|Texas Instruments Incorporated
|XWR6243
[IBIS Ver]   4.1
[File name]   xwr6243_v1.ibs
[Date]   06/24/2022
[File Rev]   1.0
[Source]
| Texas Instruments Incorporated.
| Analog-eLab Design Center, HPA
| 12500 TI Blvd
| Dallas, TX -75243
[Notes]   Revision History:
| Rev 1.0: 06/24/2022
| - Initial version of the model
|   Model names with a trailing _1p8 contain the model for 1.8V operation.
|   Model names with a trailing _3p3 contain the model for 3.3V operation.
| - C_comp although listed in numerical order of value are
|   obtained from varying PVT conditions. For PVT conditions for
|   each specific value refer the buffer description under
|   respective [Model]. IBIS model user is responsible for using
|   appropriate C_comp to simulate for Signal Integrity.
[Disclaimer]
| This model is designed as an aid for customers of Texas Instruments.
| TI and its licensors and suppliers make no warranties, either expressed
| or implied, with respect to this  model, including the warranties of
| merchantability or fitness for a particular purpose. The model is
| provided solely on an "as is" basis. The entire risk as to its quality
| and performance is with the customer.
| This model is subject to change without notice. Texas Instruments
| Incorporated is not responsible for updating this model.
[Copyright]
(C) Copyright 2022 Texas Instruments Incorporated.All rights reserved.
|  Component XWR6243ABGABL 161-pin FCBGA -ABL0161 package
|  Part # AWR6243ABGABLQ1/IWR6243ABGABL
[Component]   XWR6243ABGABL
[Manufacturer]   Texas Instruments
[Package]   |161 FCBGA -ABL0161 package
|  variable   typ   min   max
R_pkg   0.05   0.04   0.06
L_pkg   1.0nH   0.8nH   1.2nH
C_pkg   0.2pF   0.16pF   0.24pF
[Pin]   signal_name   model_name   R_pin   L_pin   C_pin
A1   VSSA   GND   NA   NA   NA
A2   VOUT_PA   NC   NA   NA   NA
A3   VSSA   GND   NA   NA   NA
A5   VSSA   GND   NA   NA   NA
A7   VSSA   GND   NA   NA   NA
A9   VSSA   GND   NA   NA   NA
A10   VOUT_14APLL   NC   NA   NA   NA
A13   VOUT_14SYNTH   NC   NA   NA   NA
A14   OSC_CLKOUT   OUT   NA   NA   NA
A15   VSSA   GND   NA   NA   NA
B1   FM_CW_SYNCIN1   NC   NA   NA   NA
B2   VOUT_PA   NC   NA   NA   NA
B3   VSSA   GND   NA   NA   NA
B4   TX1   NC   NA   NA   NA
B5   VSSA   GND   NA   NA   NA
B6   TX2   NC   NA   NA   NA
B7   VSSA   GND   NA   NA   NA
B8   TX3   NC   NA   NA   NA
B9   VSSA   GND   NA   NA   NA
B10   VBGAP   NC   NA   NA   NA
B11   VIN_18CLK   POWER   NA   NA   NA
B12   VIN_18VCO   POWER   NA   NA   NA
B13   VSSA   GND   NA   NA   NA
B14   VSSA   GND   NA   NA   NA
B15   FM_CW_CLKOUT   NC   NA   NA   NA
C1   VSSA   GND   NA   NA   NA
C2   VIN_13RF2   POWER   NA   NA   NA
C3   VSSA   GND   NA   NA   NA
C4   VSSA   GND   NA   NA   NA
C5   VSSA   GND   NA   NA   NA
C6   VSSA   GND   NA   NA   NA
C7   VSSA   GND   NA   NA   NA
C8   VSSA   GND   NA   NA   NA
C9   VSSA   GND   NA   NA   NA
C13   ANAMUX/GPADC5   NC   NA   NA   NA
C14   VSENSE/GPADC6   NC   NA   NA   NA
C15   VSSA   GND   NA   NA   NA
D1   FM_CW_SYNCOUT   NC   NA   NA   NA
D2   VIN_13RF2   POWER   NA   NA   NA
D13   VIOIN_18DIFF   POWER   NA   NA   NA
D15   FM_CW_SYNCIN2   NC   NA   NA   NA
E1   VSSA   GND   NA   NA   NA
E2   VSSA   GND   NA   NA   NA
E3   VSSA   GND   NA   NA   NA
E5   VSS   GND   NA   NA   NA
E6   VSS   GND   NA   NA   NA
E8   VSS   GND   NA   NA   NA
E10   VSS   GND   NA   NA   NA
E11   VSS   GND   NA   NA   NA
E13   VSSA   GND   NA   NA   NA
E14   CLKP   NC   NA   NA   NA
E15   VSSA   GND   NA   NA   NA
F2   RX4   NC   NA   NA   NA
F3   VSSA   GND   NA   NA   NA
F5   VIN_18BB   POWER   NA   NA   NA
F9   VSS   GND   NA   NA   NA
F11   VSS   GND   NA   NA   NA
F13   VDDIN   POWER   NA   NA   NA
F14   CLKM   NC   NA   NA   NA
G1   VSSA   GND   NA   NA   NA
G2   VSSA   GND   NA   NA   NA
G3   VSSA   GND   NA   NA   NA
G5   VIN_13RF1   POWER   NA   NA   NA
G6   VSS   GND   NA   NA   NA
G7   VSS   GND   NA   NA   NA
G8   VSS   GND   NA   NA   NA
G10   VSS   GND   NA   NA   NA
G13   Reserved   POWER   NA   NA   NA
G14   CSI2_TXM[0]   ODF1   NA   NA   NA
G15   CSI2_TXP[0]   ODF1   NA   NA   NA
H2   RX3   NC   NA   NA   NA
H3   VSSA   GND   NA   NA   NA
H5   VIN_13RF1   POWER   NA   NA   NA
H7   VSS   GND   NA   NA   NA
H9   VSS   GND   NA   NA   NA
H11   VSS   GND   NA   NA   NA
H13   TDI   IO2   NA   NA   NA
H14   CSI2_TXM[1]   ODF2   NA   NA   NA
H15   CSI2_TXP[1]   ODF2   NA   NA   NA
J1   VSSA   GND   NA   NA   NA
J2   VSSA   GND   NA   NA   NA
J3   VSSA   GND   NA   NA   NA
J5   VIN_13RF1   POWER   NA   NA   NA
J6   VSS   GND   NA   NA   NA
J7   VSS   GND   NA   NA   NA
J8   VSS   GND   NA   NA   NA
J10   VSS   GND   NA   NA   NA
J13   TDO   IO2   NA   NA   NA
J14   CSI2_CLKM   ODF1   NA   NA   NA
J15   CSI2_CLKP   ODF1   NA   NA   NA
K2   RX2   NC   NA   NA   NA
K3   VSSA   GND   NA   NA   NA
K5   VIN_18BB   POWER   NA   NA   NA
K7   VSS   GND   NA   NA   NA
K8   VSS   GND   NA   NA   NA
K9   VSS   GND   NA   NA   NA
K10   VSS   GND   NA   NA   NA
K11   VSS   GND   NA   NA   NA
K13   VIOIN_18   POWER   NA   NA   NA
K14   CSI2_TXM[2]   ODF2   NA   NA   NA
K15   CSI2_TXP[2]   ODF2   NA   NA   NA
L1   VSSA   GND   NA   NA   NA
L2   VSSA   GND   NA   NA   NA
L3   VSSA   GND   NA   NA   NA
L5   VSS   GND   NA   NA   NA
L6   VSS   GND   NA   NA   NA
L8   VSS   GND   NA   NA   NA
L10   VSS   GND   NA   NA   NA
L13   TMS   IO2   NA   NA   NA
L14   CSI2_TXM[3]   ODF2   NA   NA   NA
L15   CSI2_TXP[3]   ODF2   NA   NA   NA
M2   RX1   NC   NA   NA   NA
M3   VSSA   GND   NA   NA   NA
M13   TCK   IO2   NA   NA   NA
M14   HS_M_Debug1   NC   NA   NA   NA
M15   HS_P_Debug1   NC   NA   NA   NA
N1   VSSA   GND   NA   NA   NA
N2   VSSA   GND   NA   NA   NA
N3   VSSA   GND   NA   NA   NA
N4   GPIO[0]   IO1   NA   NA   NA
N5   RS232_RX   IO1   NA   NA   NA
N6   RS232_TX   IO1   NA   NA   NA
N7   GPIO[1]   IO1   NA   NA   NA
N8   NERROR_OUT   IOOD   NA   NA   NA
N9   MCU_CLK_OUT   IO1   NA   NA   NA
N10   SYNC_IN   IO2   NA   NA   NA
N11   VDDIN   POWER   NA   NA   NA
N12   WARM_RESET   IOOD   NA   NA   NA
N13   GPIO[2]   IO2   NA   NA   NA
N14   HS_M_Debug2   NC   NA   NA   NA
N15   HS_P_Debug2   NC   NA   NA   NA
P1   AnalogTest1/GPADC1  NC   NA   NA   NA
P2   AnalogTest2/GPADC2  NC   NA   NA   NA
P3   AnalogTest3/GPADC3  NC   NA   NA   NA
P4   Reserved   NC   NA   NA   NA
P5   MISO_1   IO1   NA   NA   NA
P6   SPI_HOST_INTR   NC   NA   NA   NA
P7   NERROR_IN   IOOD   NA   NA   NA
P8   QSPI_CS   IO1   NA   NA   NA
P9   QSPI[1]   IO1   NA   NA   NA
P10   QSPI[3]   IO1   NA   NA   NA
P11   SYNC_OUT   IO2   NA   NA   NA
P12   NRESET   NC   NA   NA   NA
P13   PMIC_CLK_OUT   IO2   NA   NA   NA
P14   VNWA   POWER   NA   NA   NA
P15   VDDIN   POWER   NA   NA   NA
R1   VSSA   GND   NA   NA   NA
R2   AnalogTest4/GPADC4  NC   NA   NA   NA
R3   Reserved   NC   NA   NA   NA
R4   Reserved   NC   NA   NA   NA
R5   Reserved   NC   NA   NA   NA
R6   VDDIN   POWER   NA   NA   NA
R7   SPI_CS_1   IO1   NA   NA   NA
R8   MOSI_1   IO1   NA   NA   NA
R9   SPI_CLK_1   IO1   NA   NA   NA
R10   QSPI_CLK   IO1   NA   NA   NA
R11   QSPI[0]   IO2   NA   NA   NA
R12   QSPI[2]   IO2   NA   NA   NA
R13   VIOIN   POWER   NA   NA   NA
R14   VIN_SRAM   POWER   NA   NA   NA
R15   VSS   GND   NA   NA   NA
[Diff Pin]   inv_pin   vdiff   tdelay_typ   tdelay_min   tdelay_max
G15   G14   0.2   NA   NA   NA
H15   H14   0.2   NA   NA   NA
J15   J14   0.2   NA   NA   NA
K15   K14   0.2   NA   NA   NA
L15   L14   0.2   NA   NA   NA
|  Component XWR6243ABGABLR 161-pin FCBGA -ABL0161 package
|  Part # AWR6243ABGABLRQ1/IWR6243ABGABLR
[Component]   XWR6243ABGABLR
[Manufacturer]   Texas Instruments
[Package]   |161 FCBGA -ABL0161 package
|  variable   typ   min   max
R_pkg   0.05   0.04   0.06
L_pkg   1.0nH   0.8nH   1.2nH
C_pkg   0.2pF   0.16pF   0.24pF
[Pin]   signal_name   model_name   R_pin   L_pin   C_pin
A1   VSSA   GND   NA   NA   NA
A2   VOUT_PA   NC   NA   NA   NA
A3   VSSA   GND   NA   NA   NA
A5   VSSA   GND   NA   NA   NA
A7   VSSA   GND   NA   NA   NA
A9   VSSA   GND   NA   NA   NA
A10   VOUT_14APLL   NC   NA   NA   NA
A13   VOUT_14SYNTH   NC   NA   NA   NA
A14   OSC_CLKOUT   OUT   NA   NA   NA
A15   VSSA   GND   NA   NA   NA
B1   FM_CW_SYNCIN1   NC   NA   NA   NA
B2   VOUT_PA   NC   NA   NA   NA
B3   VSSA   GND   NA   NA   NA
B4   TX1   NC   NA   NA   NA
B5   VSSA   GND   NA   NA   NA
B6   TX2   NC   NA   NA   NA
B7   VSSA   GND   NA   NA   NA
B8   TX3   NC   NA   NA   NA
B9   VSSA   GND   NA   NA   NA
B10   VBGAP   NC   NA   NA   NA
B11   VIN_18CLK   POWER   NA   NA   NA
B12   VIN_18VCO   POWER   NA   NA   NA
B13   VSSA   GND   NA   NA   NA
B14   VSSA   GND   NA   NA   NA
B15   FM_CW_CLKOUT   NC   NA   NA   NA
C1   VSSA   GND   NA   NA   NA
C2   VIN_13RF2   POWER   NA   NA   NA
C3   VSSA   GND   NA   NA   NA
C4   VSSA   GND   NA   NA   NA
C5   VSSA   GND   NA   NA   NA
C6   VSSA   GND   NA   NA   NA
C7   VSSA   GND   NA   NA   NA
C8   VSSA   GND   NA   NA   NA
C9   VSSA   GND   NA   NA   NA
C13   ANAMUX/GPADC5   NC   NA   NA   NA
C14   VSENSE/GPADC6   NC   NA   NA   NA
C15   VSSA   GND   NA   NA   NA
D1   FM_CW_SYNCOUT   NC   NA   NA   NA
D2   VIN_13RF2   POWER   NA   NA   NA
D13   VIOIN_18DIFF   POWER   NA   NA   NA
D15   FM_CW_SYNCIN2   NC   NA   NA   NA
E1   VSSA   GND   NA   NA   NA
E2   VSSA   GND   NA   NA   NA
E3   VSSA   GND   NA   NA   NA
E5   VSS   GND   NA   NA   NA
E6   VSS   GND   NA   NA   NA
E8   VSS   GND   NA   NA   NA
E10   VSS   GND   NA   NA   NA
E11   VSS   GND   NA   NA   NA
E13   VSSA   GND   NA   NA   NA
E14   CLKP   NC   NA   NA   NA
E15   VSSA   GND   NA   NA   NA
F2   RX4   NC   NA   NA   NA
F3   VSSA   GND   NA   NA   NA
F5   VIN_18BB   POWER   NA   NA   NA
F9   VSS   GND   NA   NA   NA
F11   VSS   GND   NA   NA   NA
F13   VDDIN   POWER   NA   NA   NA
F14   CLKM   NC   NA   NA   NA
G1   VSSA   GND   NA   NA   NA
G2   VSSA   GND   NA   NA   NA
G3   VSSA   GND   NA   NA   NA
G5   VIN_13RF1   POWER   NA   NA   NA
G6   VSS   GND   NA   NA   NA
G7   VSS   GND   NA   NA   NA
G8   VSS   GND   NA   NA   NA
G10   VSS   GND   NA   NA   NA
G13   Reserved   POWER   NA   NA   NA
G14   CSI2_TXM[0]   ODF1   NA   NA   NA
G15   CSI2_TXP[0]   ODF1   NA   NA   NA
H2   RX3   NC   NA   NA   NA
H3   VSSA   GND   NA   NA   NA
H5   VIN_13RF1   POWER   NA   NA   NA
H7   VSS   GND   NA   NA   NA
H9   VSS   GND   NA   NA   NA
H11   VSS   GND   NA   NA   NA
H13   TDI   IO2   NA   NA   NA
H14   CSI2_TXM[1]   ODF2   NA   NA   NA
H15   CSI2_TXP[1]   ODF2   NA   NA   NA
J1   VSSA   GND   NA   NA   NA
J2   VSSA   GND   NA   NA   NA
J3   VSSA   GND   NA   NA   NA
J5   VIN_13RF1   POWER   NA   NA   NA
J6   VSS   GND   NA   NA   NA
J7   VSS   GND   NA   NA   NA
J8   VSS   GND   NA   NA   NA
J10   VSS   GND   NA   NA   NA
J13   TDO   IO2   NA   NA   NA
J14   CSI2_CLKM   ODF1   NA   NA   NA
J15   CSI2_CLKP   ODF1   NA   NA   NA
K2   RX2   NC   NA   NA   NA
K3   VSSA   GND   NA   NA   NA
K5   VIN_18BB   POWER   NA   NA   NA
K7   VSS   GND   NA   NA   NA
K8   VSS   GND   NA   NA   NA
K9   VSS   GND   NA   NA   NA
K10   VSS   GND   NA   NA   NA
K11   VSS   GND   NA   NA   NA
K13   VIOIN_18   POWER   NA   NA   NA
K14   CSI2_TXM[2]   ODF2   NA   NA   NA
K15   CSI2_TXP[2]   ODF2   NA   NA   NA
L1   VSSA   GND   NA   NA   NA
L2   VSSA   GND   NA   NA   NA
L3   VSSA   GND   NA   NA   NA
L5   VSS   GND   NA   NA   NA
L6   VSS   GND   NA   NA   NA
L8   VSS   GND   NA   NA   NA
L10   VSS   GND   NA   NA   NA
L13   TMS   IO2   NA   NA   NA
L14   CSI2_TXM[3]   ODF2   NA   NA   NA
L15   CSI2_TXP[3]   ODF2   NA   NA   NA
M2   RX1   NC   NA   NA   NA
M3   VSSA   GND   NA   NA   NA
M13   TCK   IO2   NA   NA   NA
M14   HS_M_Debug1   NC   NA   NA   NA
M15   HS_P_Debug1   NC   NA   NA   NA
N1   VSSA   GND   NA   NA   NA
N2   VSSA   GND   NA   NA   NA
N3   VSSA   GND   NA   NA   NA
N4   GPIO[0]   IO1   NA   NA   NA
N5   RS232_RX   IO1   NA   NA   NA
N6   RS232_TX   IO1   NA   NA   NA
N7   GPIO[1]   IO1   NA   NA   NA
N8   NERROR_OUT   IOOD   NA   NA   NA
N9   MCU_CLK_OUT   IO1   NA   NA   NA
N10   SYNC_IN   IO2   NA   NA   NA
N11   VDDIN   POWER   NA   NA   NA
N12   WARM_RESET   IOOD   NA   NA   NA
N13   GPIO[2]   IO2   NA   NA   NA
N14   HS_M_Debug2   NC   NA   NA   NA
N15   HS_P_Debug2   NC   NA   NA   NA
P1   AnalogTest1/GPADC1  NC   NA   NA   NA
P2   AnalogTest2/GPADC2  NC   NA   NA   NA
P3   AnalogTest3/GPADC3  NC   NA   NA   NA
P4   Reserved   NC   NA   NA   NA
P5   MISO_1   IO1   NA   NA   NA
P6   SPI_HOST_INTR   NC   NA   NA   NA
P7   NERROR_IN   IOOD   NA   NA   NA
P8   QSPI_CS   IO1   NA   NA   NA
P9   QSPI[1]   IO1   NA   NA   NA
P10   QSPI[3]   IO1   NA   NA   NA
P11   SYNC_OUT   IO2   NA   NA   NA
P12   NRESET   NC   NA   NA   NA
P13   PMIC_CLK_OUT   IO2   NA   NA   NA
P14   VNWA   POWER   NA   NA   NA
P15   VDDIN   POWER   NA   NA   NA
R1   VSSA   GND   NA   NA   NA
R2   AnalogTest4/GPADC4  NC   NA   NA   NA
R3   Reserved   NC   NA   NA   NA
R4   Reserved   NC   NA   NA   NA
R5   Reserved   NC   NA   NA   NA
R6   VDDIN   POWER   NA   NA   NA
R7   SPI_CS_1   IO1   NA   NA   NA
R8   MOSI_1   IO1   NA   NA   NA
R9   SPI_CLK_1   IO1   NA   NA   NA
R10   QSPI_CLK   IO1   NA   NA   NA
R11   QSPI[0]   IO2   NA   NA   NA
R12   QSPI[2]   IO2   NA   NA   NA
R13   VIOIN   POWER   NA   NA   NA
R14   VIN_SRAM   POWER   NA   NA   NA
R15   VSS   GND   NA   NA   NA
[Diff Pin]   inv_pin   vdiff   tdelay_typ   tdelay_min   tdelay_max
G15   G14   0.2   NA   NA   NA
H15   H14   0.2   NA   NA   NA
J15   J14   0.2   NA   NA   NA
K15   K14   0.2   NA   NA   NA
L15   L14   0.2   NA   NA   NA
| Model IOOD
[Model Selector] IOOD
|SC1 IS A SLEW RATE CONTROL PIN
|5% SUPPLY VARIATION MODES WITH 1.8V NOM SUPPLY
IOOD_V_PUPDOFF_5P_SC1_1P8  Cell operated at 1.8(nom)
|IOOD_V_PUPDOFF_5P_SC1_1P8; BUFFER WITH WEAK PULUP/PULLDOWN OFF AT 5% SUPPLY
|VARIATION WITH SC1=1 MEANING SLOW MODE OF OPERATION
IOOD_V_PD_ON_5P_!SC1_1P8  Cell operated at 1.8(nom)
|IOOD_V_PD_ON_5P_!SC1_1P8; BUFFER WITH WEAK_PULLDOWN_ON AT 5% SUPPLY
|VARIATION WITH SC1=0 MEANING FAST MODE OF OPERATION
IOOD_V_PD_ON_5P_SC1_1P8  Cell operated at 1.8(nom)
|IOOD_V_PD_ON_5P_SC1_1P8; BUFFER WITH WEAK_PULLDOWN_ON AT 5% SUPPLY
|VARIATION WITH SC1=1 MEANING SLOW MODE OF OPERATION
IOOD_V_PU_ON_5P_!SC1_1P8  Cell operated at 1.8(nom)
|IOOD_V_PU_ON_5P_!SC1_1P8; BUFFER WITH WEAK_PULLUP_ON AT 5% SUPPLY
|VARIATION WITH SC1=0 MEANING FAST MODE OF OPERATION
IOOD_V_PUPDOFF_5P_!SC1_1P8  Cell operated at 1.8(nom)
|IOOD_V_PUPDOFF_5P_!SC1_1P8; BUFFER WITH WEAK PULUP/PULLDOWN OFF AT 5% SUPPLY
|VARIATION WITH SC1=0 MEANING FAST MODE OF OPERATION
IOOD_V_PU_ON_5P_SC1_1P8  Cell operated at 1.8(nom)
|IOOD_V_PU_ON_5P_SC1_1P8; BUFFER WITH WEAK_PULLUP_ON AT 5% SUPPLY
|VARIATION WITH SC1=1 MEANING SLOW MODE OF OPERATION
|5% SUPPLY VARIATION MODES WITH 3.3V NOM SUPPLY
IOOD_V_PUPDOFF_5P_SC1_3P3  Cell operated at 3.3(nom)
|IOOD_V_PUPDOFF_5P_SC1_3P3; BUFFER WITH WEAK PULUP/PULLDOWN OFF AT 5% SUPPLY
|VARIATION WITH SC1=1 MEANING SLOW MODE OF OPERATION
IOOD_V_PD_ON_5P_!SC1_3P3  Cell operated at 3.3(nom)
|IOOD_V_PD_ON_5P_!SC1_3P3; BUFFER WITH WEAK_PULLDOWN_ON AT 5% SUPPLY
|VARIATION WITH SC1=0 MEANING FAST MODE OF OPERATION
IOOD_V_PD_ON_5P_SC1_3P3  Cell operated at 3.3(nom)
|IOOD_V_PD_ON_5P_SC1_3P3; BUFFER WITH WEAK_PULLDOWN_ON AT 5% SUPPLY
|VARIATION WITH SC1=1 MEANING SLOW MODE OF OPERATION
IOOD_V_PU_ON_5P_!SC1_3P3  Cell operated at 3.3(nom)
|IOOD_V_PU_ON_5P_!SC1_3P3; BUFFER WITH WEAK_PULLUP_ON AT 5% SUPPLY
|VARIATION WITH SC1=0 MEANING FAST MODE OF OPERATION
IOOD_V_PUPDOFF_5P_!SC1_3P3  Cell operated at 3.3(nom)
|IOOD_V_PUPDOFF_5P_!SC1_3P3; BUFFER WITH WEAK PULUP/PULLDOWN OFF AT 5% SUPPLY
|VARIATION WITH SC1=0 MEANING FAST MODE OF OPERATION
IOOD_V_PU_ON_5P_SC1_3P3  Cell operated at 3.3(nom)
|IOOD_V_PU_ON_5P_SC1_3P3; BUFFER WITH WEAK_PULLUP_ON AT 5% SUPPLY
|VARIATION WITH SC1=1 MEANING SLOW MODE OF OPERATION
| 10% SUPPLY VARIATION MODES WITH 1.8V NOM SUPPLY
IOOD_V_PUPDOFF_10P_SC1_1P8  Cell operated at 1.8(nom)
|IOOD_V_PUPDOFF_10P_SC1_1P8; BUFFER WITH WEAK PULUP/PULLDOWN OFF AT 10% SUPPLY
|VARIATION WITH SC1=1 MEANING SLOW MODE OF OPERATION
IOOD_V_PD_ON_10P_!SC1_1P8  Cell operated at 1.8(nom)
|IOOD_V_PD_ON_10P_!SC1_1P8; BUFFER WITH WEAK_PULLDOWN_ON AT 10% SUPPLY
|VARIATION WITH SC1=0 MEANING FAST MODE OF OPERATION
IOOD_V_PD_ON_10P_SC1_1P8  Cell operated at 1.8(nom)
|IOOD_V_PD_ON_10P_SC1_1P8; BUFFER WITH WEAK_PULLDOWN_ON AT 10% SUPPLY
|VARIATION WITH SC1=1 MEANING SLOW MODE OF OPERATION
IOOD_V_PU_ON_10P_!SC1_1P8  Cell operated at 1.8(nom)
|IOOD_V_PU_ON_10P_!SC1_1P8; BUFFER WITH WEAK_PULLUP_ON AT 10% SUPPLY
|VARIATION WITH SC1=0 MEANING FAST MODE OF OPERATION
IOOD_V_PUPDOFF_10P_!SC1_1P8  Cell operated at 1.8(nom)
|IOOD_V_PUPDOFF_10P_!SC1_1P8; BUFFER WITH WEAK PULUP/PULLDOWN OFF AT 10% SUPPLY
|VARIATION WITH SC1=0 MEANING FAST MODE OF OPERATION
IOOD_V_PU_ON_10P_SC1_1P8  Cell operated at 1.8(nom)
|IOOD_V_PU_ON_10P_SC1_1P8; BUFFER WITH WEAK_PULLUP_ON AT 10% SUPPLY
|VARIATION WITH SC1=1 MEANING SLOW MODE OF OPERATION
| 10% SUPPLY VARIATION MODES WITH 3.3V NOM SUPPLY
IOOD_V_PUPDOFF_10P_SC1_3P3  Cell operated at 3.3(nom)
|IOOD_V_PUPDOFF_10P_SC1_3P3; BUFFER WITH WEAK PULUP/PULLDOWN OFF AT 10% SUPPLY
|VARIATION WITH SC1=1 MEANING SLOW MODE OF OPERATION
IOOD_V_PD_ON_10P_!SC1_3P3  Cell operated at 3.3(nom)
|IOOD_V_PD_ON_10P_!SC1_3P3; BUFFER WITH WEAK_PULLDOWN_ON 10% SUPPLY
|VARIATION WITH SC1=0 MEANING FAST MODE OF OPERATION
IOOD_V_PD_ON_10P_SC1_3P3  Cell operated at 3.3(nom)
|IOOD_V_PD_ON_10P_SC1_3P3; BUFFER WITH WEAK_PULLDOWN_ON AT 10% SUPPLY
|VARIATION WITH SC1=1 MEANING SLOW MODE OF OPERATION
IOOD_V_PU_ON_10P_!SC1_3P3  Cell operated at 3.3(nom)
|IOOD_V_PU_ON_10P_!SC1_3P3; BUFFER WITH WEAK_PULLUP_ON AT 10% SUPPLY
|VARIATION WITH SC1=0 MEANING FAST MODE OF OPERATION
IOOD_V_PUPDOFF_10P_!SC1_3P3  Cell operated at 3.3(nom)
|IOOD_V_PUPDOFF_10P_!SC1_3P3; BUFFER WITH WEAK PULUP/PULLDOWN OFF AT 10% SUPPLY
|VARIATION WITH SC1=0 MEANING FAST MODE OF OPERATION
IOOD_V_PU_ON_10P_SC1_3P3  Cell operated at 3.3(nom)
|IOOD_V_PU_ON_10P_SC1_3P3; BUFFER WITH WEAK_PULLUP_ON AT 10% SUPPLY
|VARIATION WITH SC1=1 MEANING SLOW MODE OF OPERATION
| Model IO1
[Model Selector] IO1
|SC1 IS A SLEW RATE CONTROL PIN
|5% SUPPLY VARIATION MODES WITH 1.8V NOM SUPPLY
IO1_V_PUPDOFF_5P_SC1_1P8  Cell operated at 1.8(nom)
|IO1_V_PUPDOFF_5P_SC1_1P8; BUFFER WITH WEAK PULUP/PULLDOWN OFF AT 5% SUPPLY
|VARIATION WITH SC1=1 MEANING SLOW MODE OF OPERATION
IO1_V_PD_ON_5P_!SC1_1P8  Cell operated at 1.8(nom)
|IO1_V_PD_ON_5P_!SC1_1P8; BUFFER WITH WEAK_PULLDOWN_ON AT 5% SUPPLY
|VARIATION WITH SC1=0 MEANING FAST MODE OF OPERATION
IO1_V_PD_ON_5P_SC1_1P8  Cell operated at 1.8(nom)
|IO1_V_PD_ON_5P_SC1_1P8; BUFFER WITH WEAK_PULLDOWN_ON AT 5% SUPPLY
|VARIATION WITH SC1=1 MEANING SLOW MODE OF OPERATION
IO1_V_PU_ON_5P_!SC1_1P8  Cell operated at 1.8(nom)
|IO1_V_PU_ON_5P_!SC1_1P8; BUFFER WITH WEAK_PULLUP_ON AT 5% SUPPLY
|VARIATION WITH SC1=0 MEANING FAST MODE OF OPERATION
IO1_V_PUPDOFF_5P_!SC1_1P8  Cell operated at 1.8(nom)
|IO1_V_PUPDOFF_5P_!SC1_1P8; BUFFER WITH WEAK PULUP/PULLDOWN OFF AT 5% SUPPLY
|VARIATION WITH SC1=0 MEANING FAST MODE OF OPERATION
IO1_V_PU_ON_5P_SC1_1P8  Cell operated at 1.8(nom)
|IO1_V_PU_ON_5P_SC1_1P8; BUFFER WITH WEAK_PULLUP_ON AT 5% SUPPLY
|VARIATION WITH SC1=1 MEANING SLOW MODE OF OPERATION
|5% SUPPLY VARIATION MODES WITH 3.3V NOM SUPPLY
IO1_V_PUPDOFF_5P_SC1_3P3  Cell operated at 3.3(nom)
|IO1_V_PUPDOFF_5P_SC1_3P3; BUFFER WITH WEAK PULUP/PULLDOWN OFF AT 5% SUPPLY
|VARIATION WITH SC1=1 MEANING SLOW MODE OF OPERATION
IO1_V_PD_ON_5P_!SC1_3P3  Cell operated at 3.3(nom)
|IO1_V_PD_ON_5P_!SC1_3P3; BUFFER WITH WEAK_PULLDOWN_ON AT 5% SUPPLY
|VARIATION WITH SC1=0 MEANING FAST MODE OF OPERATION
IO1_V_PD_ON_5P_SC1_3P3  Cell operated at 3.3(nom)
|IO1_V_PD_ON_5P_SC1_3P3; BUFFER WITH WEAK_PULLDOWN_ON AT 5% SUPPLY
|VARIATION WITH SC1=1 MEANING SLOW MODE OF OPERATION
IO1_V_PU_ON_5P_!SC1_3P3  Cell operated at 3.3(nom)
|IO1_V_PU_ON_5P_!SC1_3P3; BUFFER WITH WEAK_PULLUP_ON AT 5% SUPPLY
|VARIATION WITH SC1=0 MEANING FAST MODE OF OPERATION
IO1_V_PUPDOFF_5P_!SC1_3P3  Cell operated at 3.3(nom)
|IO1_V_PUPDOFF_5P_!SC1_3P3; BUFFER WITH WEAK PULUP/PULLDOWN OFF AT 5% SUPPLY
|VARIATION WITH SC1=0 MEANING FAST MODE OF OPERATION
IO1_V_PU_ON_5P_SC1_3P3  Cell operated at 3.3(nom)
|IO1_V_PU_ON_5P_SC1_3P3; BUFFER WITH WEAK_PULLUP_ON AT 5% SUPPLY
|VARIATION WITH SC1=1 MEANING SLOW MODE OF OPERATION
| 10% SUPPLY VARIATION MODES WITH 1.8V NOM SUPPLY
IO1_V_PUPDOFF_10P_SC1_1P8  Cell operated at 1.8(nom)
|IO1_V_PUPDOFF_10P_SC1_1P8; BUFFER WITH WEAK PULUP/PULLDOWN OFF AT 10% SUPPLY
|VARIATION WITH SC1=1 MEANING SLOW MODE OF OPERATION
IO1_V_PD_ON_10P_!SC1_1P8  Cell operated at 1.8(nom)
|IO1_V_PD_ON_10P_!SC1_1P8; BUFFER WITH WEAK_PULLDOWN_ON AT 10% SUPPLY
|VARIATION WITH SC1=0 MEANING FAST MODE OF OPERATION
IO1_V_PD_ON_10P_SC1_1P8  Cell operated at 1.8(nom)
|IO1_V_PD_ON_10P_SC1_1P8; BUFFER WITH WEAK_PULLDOWN_ON AT 10% SUPPLY
|VARIATION WITH SC1=1 MEANING SLOW MODE OF OPERATION
IO1_V_PU_ON_10P_!SC1_1P8  Cell operated at 1.8(nom)
|IO1_V_PU_ON_10P_!SC1_1P8; BUFFER WITH WEAK_PULLUP_ON AT 10% SUPPLY
|VARIATION WITH SC1=0 MEANING FAST MODE OF OPERATION
IO1_V_PUPDOFF_10P_!SC1_1P8  Cell operated at 1.8(nom)
|IO1_V_PUPDOFF_10P_!SC1_1P8; BUFFER WITH WEAK PULUP/PULLDOWN OFF AT 10% SUPPLY
|VARIATION WITH SC1=0 MEANING FAST MODE OF OPERATION
IO1_V_PU_ON_10P_SC1_1P8  Cell operated at 1.8(nom)
|IO1_V_PU_ON_10P_SC1_1P8; BUFFER WITH WEAK_PULLUP_ON AT 10% SUPPLY
|VARIATION WITH SC1=1 MEANING SLOW MODE OF OPERATION
| 10% SUPPLY VARIATION MODES WITH 3.3V NOM SUPPLY
IO1_V_PUPDOFF_10P_SC1_3P3  Cell operated at 3.3(nom)
|IO1_V_PUPDOFF_10P_SC1_3P3; BUFFER WITH WEAK PULUP/PULLDOWN OFF AT 10% SUPPLY
|VARIATION WITH SC1=1 MEANING SLOW MODE OF OPERATION
IO1_V_PD_ON_10P_!SC1_3P3  Cell operated at 3.3(nom)
|IO1_V_PD_ON_10P_!SC1_3P3; BUFFER WITH WEAK_PULLDOWN_ON 10% SUPPLY
|VARIATION WITH SC1=0 MEANING FAST MODE OF OPERATION
IO1_V_PD_ON_10P_SC1_3P3  Cell operated at 3.3(nom)
|IO1_V_PD_ON_10P_SC1_3P3; BUFFER WITH WEAK_PULLDOWN_ON AT 10% SUPPLY
|VARIATION WITH SC1=1 MEANING SLOW MODE OF OPERATION
IO1_V_PU_ON_10P_!SC1_3P3  Cell operated at 3.3(nom)
|IO1_V_PU_ON_10P_!SC1_3P3; BUFFER WITH WEAK_PULLUP_ON AT 10% SUPPLY
|VARIATION WITH SC1=0 MEANING FAST MODE OF OPERATION
IO1_V_PUPDOFF_10P_!SC1_3P3  Cell operated at 3.3(nom)
|IO1_V_PUPDOFF_10P_!SC1_3P3; BUFFER WITH WEAK PULUP/PULLDOWN OFF AT 10% SUPPLY
|VARIATION WITH SC1=0 MEANING FAST MODE OF OPERATION
IO1_V_PU_ON_10P_SC1_3P3  Cell operated at 3.3(nom)
|IO1_V_PU_ON_10P_SC1_3P3; BUFFER WITH WEAK_PULLUP_ON AT 10% SUPPLY
|VARIATION WITH SC1=1 MEANING SLOW MODE OF OPERATION
| Model IO2
[Model Selector] IO2
|SC1 IS A SLEW RATE CONTROL PIN
|5% SUPPLY VARIATION MODES WITH 1.8V NOM SUPPLY
IO2_H_PUPDOFF_5P_SC1_1P8  Cell operated at 1.8(nom)
|IO2_H_PUPDOFF_5P_SC1_1P8; BUFFER WITH WEAK PULUP/PULLDOWN OFF AT 5% SUPPLY
|VARIATION WITH SC1=1 MEANING SLOW MODE OF OPERATION
IO2_H_PD_ON_5P_!SC1_1P8  Cell operated at 1.8(nom)
|IO2_H_PD_ON_5P_!SC1_1P8; BUFFER WITH WEAK_PULLDOWN_ON AT 5% SUPPLY
|VARIATION WITH SC1=0 MEANING FAST MODE OF OPERATION
IO2_H_PD_ON_5P_SC1_1P8  Cell operated at 1.8(nom)
|IO2_H_PD_ON_5P_SC1_1P8; BUFFER WITH WEAK_PULLDOWN_ON AT 5% SUPPLY
|VARIATION WITH SC1=1 MEANING SLOW MODE OF OPERATION
IO2_H_PU_ON_5P_!SC1_1P8  Cell operated at 1.8(nom)
|IO2_H_PU_ON_5P_!SC1_1P8; BUFFER WITH WEAK_PULLUP_ON AT 5% SUPPLY
|VARIATION WITH SC1=0 MEANING FAST MODE OF OPERATION
IO2_H_PUPDOFF_5P_!SC1_1P8  Cell operated at 1.8(nom)
|IO2_H_PUPDOFF_5P_!SC1_1P8; BUFFER WITH WEAK PULUP/PULLDOWN OFF AT 5% SUPPLY
|VARIATION WITH SC1=0 MEANING FAST MODE OF OPERATION
IO2_H_PU_ON_5P_SC1_1P8  Cell operated at 1.8(nom)
|IO2_H_PU_ON_5P_SC1_1P8; BUFFER WITH WEAK_PULLUP_ON AT 5% SUPPLY
|VARIATION WITH SC1=1 MEANING SLOW MODE OF OPERATION
|5% SUPPLY VARIATION MODES WITH 3.3V NOM SUPPLY
IO2_H_PUPDOFF_5P_SC1_3P3  Cell operated at 3.3(nom)
|IO2_H_PUPDOFF_5P_SC1_3P3; BUFFER WITH WEAK PULUP/PULLDOWN OFF AT 5% SUPPLY
|VARIATION WITH SC1=1 MEANING SLOW MODE OF OPERATION
IO2_H_PD_ON_5P_!SC1_3P3  Cell operated at 3.3(nom)
|IO2_H_PD_ON_5P_!SC1_3P3; BUFFER WITH WEAK_PULLDOWN_ON AT 5% SUPPLY
|VARIATION WITH SC1=0 MEANING FAST MODE OF OPERATION
IO2_H_PD_ON_5P_SC1_3P3  Cell operated at 3.3(nom)
|IO2_H_PD_ON_5P_SC1_3P3; BUFFER WITH WEAK_PULLDOWN_ON AT 5% SUPPLY
|VARIATION WITH SC1=1 MEANING SLOW MODE OF OPERATION
IO2_H_PU_ON_5P_!SC1_3P3  Cell operated at 3.3(nom)
|IO2_H_PU_ON_5P_!SC1_3P3; BUFFER WITH WEAK_PULLUP_ON AT 5% SUPPLY
|VARIATION WITH SC1=0 MEANING FAST MODE OF OPERATION
IO2_H_PUPDOFF_5P_!SC1_3P3  Cell operated at 3.3(nom)
|IO2_H_PUPDOFF_5P_!SC1_3P3; BUFFER WITH WEAK PULUP/PULLDOWN OFF AT 5% SUPPLY
|VARIATION WITH SC1=0 MEANING FAST MODE OF OPERATION
IO2_H_PU_ON_5P_SC1_3P3  Cell operated at 3.3(nom)
|IO2_H_PU_ON_5P_SC1_3P3; BUFFER WITH WEAK_PULLUP_ON AT 5% SUPPLY
|VARIATION WITH SC1=1 MEANING SLOW MODE OF OPERATION
| 10% SUPPLY VARIATION MODES WITH 1.8V NOM SUPPLY
IO2_H_PUPDOFF_10P_SC1_1P8  Cell operated at 1.8(nom)
|IO2_H_PUPDOFF_10P_SC1_1P8; BUFFER WITH WEAK PULUP/PULLDOWN OFF AT 10% SUPPLY
|VARIATION WITH SC1=1 MEANING SLOW MODE OF OPERATION
IO2_H_PD_ON_10P_!SC1_1P8  Cell operated at 1.8(nom)
|IO2_H_PD_ON_10P_!SC1_1P8; BUFFER WITH WEAK_PULLDOWN_ON AT 10% SUPPLY
|VARIATION WITH SC1=0 MEANING FAST MODE OF OPERATION
IO2_H_PD_ON_10P_SC1_1P8  Cell operated at 1.8(nom)
|IO2_H_PD_ON_10P_SC1_1P8; BUFFER WITH WEAK_PULLDOWN_ON AT 10% SUPPLY
|VARIATION WITH SC1=1 MEANING SLOW MODE OF OPERATION
IO2_H_PU_ON_10P_!SC1_1P8  Cell operated at 1.8(nom)
|IO2_H_PU_ON_10P_!SC1_1P8; BUFFER WITH WEAK_PULLUP_ON AT 10% SUPPLY
|VARIATION WITH SC1=0 MEANING FAST MODE OF OPERATION
IO2_H_PUPDOFF_10P_!SC1_1P8  Cell operated at 1.8(nom)
|IO2_H_PUPDOFF_10P_!SC1_1P8; BUFFER WITH WEAK PULUP/PULLDOWN OFF AT 10% SUPPLY
|VARIATION WITH SC1=0 MEANING FAST MODE OF OPERATION
IO2_H_PU_ON_10P_SC1_1P8  Cell operated at 1.8(nom)
|IO2_H_PU_ON_10P_SC1_1P8; BUFFER WITH WEAK_PULLUP_ON AT 10% SUPPLY
|VARIATION WITH SC1=1 MEANING SLOW MODE OF OPERATION
| 10% SUPPLY VARIATION MODES WITH 3.3V NOM SUPPLY
IO2_H_PUPDOFF_10P_SC1_3P3  Cell operated at 3.3(nom)
|IO2_H_PUPDOFF_10P_SC1_3P3; BUFFER WITH WEAK PULUP/PULLDOWN OFF AT 10% SUPPLY
|VARIATION WITH SC1=1 MEANING SLOW MODE OF OPERATION
IO2_H_PD_ON_10P_!SC1_3P3  Cell operated at 3.3(nom)
|IO2_H_PD_ON_10P_!SC1_3P3; BUFFER WITH WEAK_PULLDOWN_ON 10% SUPPLY
|VARIATION WITH SC1=0 MEANING FAST MODE OF OPERATION
IO2_H_PD_ON_10P_SC1_3P3  Cell operated at 3.3(nom)
|IO2_H_PD_ON_10P_SC1_3P3; BUFFER WITH WEAK_PULLDOWN_ON AT 10% SUPPLY
|VARIATION WITH SC1=1 MEANING SLOW MODE OF OPERATION
IO2_H_PU_ON_10P_!SC1_3P3  Cell operated at 3.3(nom)
|IO2_H_PU_ON_10P_!SC1_3P3; BUFFER WITH WEAK_PULLUP_ON AT 10% SUPPLY
|VARIATION WITH SC1=0 MEANING FAST MODE OF OPERATION
IO2_H_PUPDOFF_10P_!SC1_3P3  Cell operated at 3.3(nom)
|IO2_H_PUPDOFF_10P_!SC1_3P3; BUFFER WITH WEAK PULUP/PULLDOWN OFF AT 10% SUPPLY
|VARIATION WITH SC1=0 MEANING FAST MODE OF OPERATION
IO2_H_PU_ON_10P_SC1_3P3  Cell operated at 3.3(nom)
|IO2_H_PU_ON_10P_SC1_3P3; BUFFER WITH WEAK_PULLUP_ON AT 10% SUPPLY
|VARIATION WITH SC1=1 MEANING SLOW MODE OF OPERATION
| Model ODF
[Model Selector] ODF1
ODF_CORE_HSTX Cell Operated at high speed Transmitter
|ODF_CORE_HSTX; CSI2_CLKM, CSI2_CLKP, CSI2_TXM[0], CSI2_TXP[0],
|HIGH SPEED Transmitter
ODF_CORE_LPCD Cell operated at low power Contention Detection
|ODF_CORE_LPCD; CSI2_CLKM, CSI2_CLKP, CSI2_TXM[0], CSI2_TXP[0],
|LOWER POWER Contention Detection
ODF_CORE_LPRX Cell operated at low power Receiver
|ODF_CORE_LPRX; CSI2_CLKM, CSI2_CLKP, CSI2_TXM[0], CSI2_TXP[0],
|LOW POWER Receiver
ODF_CORE_LPTX Cell operated at low power Transmitter
|ODF_CORE_LPTX; CSI2_CLKM, CSI2_CLKP, CSI2_TXM[0], CSI2_TXP[0],
|LOW POWER Transmitter
ODF_CORE_ULPRX Cell operated at ultra low power Receiver
|ODF_CORE_ULPRX; CSI2_CLKM, CSI2_CLKP, CSI2_TXM[0], CSI2_TXP[0],
|ULTRA LOW POWER Receiver
[Model Selector] ODF2
ODF_ADDON_HSTX Cell Operated at high speed Transmitter
|ODF_ADDON_HSTX; CSI2_TXM[1], CSI2_TXP[1], CSI2_TXP[2], CSI2_TXM[2], CSI2_TXM[3], CSI2_TXP[3]],
|HIGH SPEED Transmitter
ODF_ADDON_LPCD Cell operated at low power Contention Detection
|ODF_ADDON_LPCD; CSI2_TXM[1], CSI2_TXP[1], CSI2_TXP[2], CSI2_TXM[2], CSI2_TXM[3], CSI2_TXP[3]],
|LOWER POWER Contention Detection
ODF_ADDON_LPRX Cell operated at low power Receiver
|ODF_ADDON_LPRX; CSI2_TXM[1], CSI2_TXP[1], CSI2_TXP[2], CSI2_TXM[2], CSI2_TXM[3], CSI2_TXP[3]],
|LOWER POWER Receiver
ODF_ADDON_LPTX Cell operated at low power Transmitter
|ODF_ADDON_LPTX; CSI2_TXM[1], CSI2_TXP[1], CSI2_TXP[2], CSI2_TXM[2], CSI2_TXM[3], CSI2_TXP[3]],
|LOWER POWER Transmitter
ODF_ADDON_ULPRX Cell operated at ultra low power Receiver
[Define Package Model]   xwr6243
[Manufacturer]   TI
[OEM]   TI
[Description]   Package
|[Number of Sections]   1
[Number of Pins]   81
[Pin Numbers]
|[Pin Name]  Net Number   Net Name   Net's All Pins
F13	|   1   VDDIN
	|N11
	|P15
	|R6
R13	|	2	VIOIN	R13
K13	|	3	VIOIN_18	K13
P1	|	4	AnalogTest1/GPADC1	P1
P2	|	5	AnalogTest2/GPADC2	P2
P3	|	6	AnalogTest3/GPADC3	P3
R2	|	7	AnalogTest4/GPADC4	R2
C13	|	8	ANAMUX/GPADC5	C13
F14	|	9	CLKM	F14
E14	|	10	CLKP	E14
B15	|	11	FM_CW_CLKOUT	B15
B1	|	12	FM_CW_SYNCIN1	B1
	|D15
D1	|	13	FM_CW_SYNCOUT	D1
N4	|	14	GPIO[0]	N4
N7	|	15	GPIO[1]	N7
N13	|	16	GPIO[2]	N13
J14	|	17	LVDS_CLKM	J14
J15	|	18	LVDS_CLKP	J15
M14	|	19	LVDS_FRCLKM	M14
M15	|	20	LVDS_FRCLKP	M15
G14	|	21	LVDS_TXM[0]	G14
H14	|	22	LVDS_TXM[1]	H14
K14	|	23	LVDS_TXM[2]	K14
L14	|	24	LVDS_TXM[3]	L14
G15	|	25	LVDS_TXP[0]	G15
H15	|	26	LVDS_TXP[1]	H15
K15	|	27	LVDS_TXP[2]	K15
L15	|	28	LVDS_TXP[3]	L15
N14	|	29	LVDS_VALIDM	N14
N15	|	30	LVDS_VALIDP	N15
N9	|	31	MCU_CLK_OUT	N9
P5	|	32	MISO_1	P5
P4	|	33	Reserved	P4
R8	|	34	MOSI_1	R8
R3	|	35	Reserved	R3
P7	|	36	NERROR_IN	P7
N8	|	37	NERROR_OUT	N8
P12	|	38	NRESET	P12
A14	|	39	OSC_CLKOUT	A14
P13	|	40	PMIC_CLK_OUT	P13
R11	|	41	QSPI[0]	R11
P9	|	42	QSPI[1]	P9
R12	|	43	QSPI[2]	R12
P10	|	44	QSPI[3]	P10
R10	|	45	QSPI_CLK	R10
P8	|	46	QSPI_CS	P8
N5	|	47	RS232_RX	N5
N6	|	48	RS232_TX	N6
M2	|	49	RX1	M2
K2	|	50	RX2	K2
H2	|	51	RX3	H2
F2	|	52	RX4	F2
R9	|	53	SPI_CLK_1	R9
R5	|	54	Reserved	R5
R7	|	55	SPI_CS_1	R7
R4	|	56	Reserved	R4
P6	|	57	SPI_HOST_INTR_1	P6
N10	|	58	SYNC_IN	N10
P11	|	59	SYNC_OUT	P11
M13	|	60	TCK	M13
H13	|	61	TDI	H13
J13	|	62	TDO	J13
L13	|	63	TMS	L13
B4	|	64	TX1	B4
B6	|	65	TX2	B6
B8	|	66	TX3	B8
B10	|	67	VBGAP	B10
G5	|	68	VIN_13RF1	G5
	|H5
	|J5
C2	|	69	VIN_13RF2	C2
	|D2
F5	|	70	VIN_18BB	F5
	|K5
B11	|	71	VIN_18CLK	B11
B12	|	72	VIN_18VCO	B12
R14	|	73	VIN_SRAM	R14
D13	|	74	VIOIN_18DIFF	D13
P14	|	75	VNWA	P14
A10	|	76	VOUT_14APLL	A10
A13	|	77	VOUT_14SYNTH	A13
A2	|	78	VOUT_PA	A2
	|B2
G13	|	79	VPP	G13
C14	|	80	VSENSE/GPADC6	C14
N12	|	81	WARM_RESET	N12
[Model Data]
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[End Model Data]
[End Package Model]
| Models and submodels in the file (83): IOOD_V_PUPDOFF_5P_SC1_1P8 (I/O_open_drain), IOOD_V_PD_ON_5P_!SC1_1P8 (I/O_open_drain), IOOD_V_PD_ON_5P_SC1_1P8 (I/O_open_drain), IOOD_V_PU_ON_5P_!SC1_1P8 (I/O_open_drain), IOOD_V_PUPDOFF_5P_!SC1_1P8 (I/O_open_drain), IOOD_V_PU_ON_5P_SC1_1P8 (I/O_open_drain), IOOD_V_PUPDOFF_5P_SC1_3P3 (I/O_open_drain), IOOD_V_PD_ON_5P_!SC1_3P3 (I/O_open_drain), IOOD_V_PD_ON_5P_SC1_3P3 (I/O_open_drain), IOOD_V_PU_ON_5P_!SC1_3P3 (I/O_open_drain), IOOD_V_PUPDOFF_5P_!SC1_3P3 (I/O_open_drain), IOOD_V_PU_ON_5P_SC1_3P3 (I/O_open_drain), IOOD_V_PUPDOFF_10P_SC1_1P8 (I/O_open_drain), IOOD_V_PD_ON_10P_!SC1_1P8 (I/O_open_drain), IOOD_V_PD_ON_10P_SC1_1P8 (I/O_open_drain), IOOD_V_PU_ON_10P_!SC1_1P8 (I/O_open_drain), IOOD_V_PUPDOFF_10P_!SC1_1P8 (I/O_open_drain), IOOD_V_PU_ON_10P_SC1_1P8 (I/O_open_drain), IOOD_V_PUPDOFF_10P_SC1_3P3 (I/O_open_drain), IOOD_V_PD_ON_10P_!SC1_3P3 (I/O_open_drain), IOOD_V_PD_ON_10P_SC1_3P3 (I/O_open_drain), IOOD_V_PU_ON_10P_!SC1_3P3 (I/O_open_drain), IOOD_V_PUPDOFF_10P_!SC1_3P3 (I/O_open_drain), IOOD_V_PU_ON_10P_SC1_3P3 (I/O_open_drain), IO1_V_PUPDOFF_5P_SC1_1P8 (I/O), IO1_V_PD_ON_5P_!SC1_1P8 (I/O), IO1_V_PD_ON_5P_SC1_1P8 (I/O), IO1_V_PU_ON_5P_!SC1_1P8 (I/O), IO1_V_PUPDOFF_5P_!SC1_1P8 (I/O), IO1_V_PU_ON_5P_SC1_1P8 (I/O), IO1_V_PUPDOFF_5P_SC1_3P3 (I/O), IO1_V_PD_ON_5P_!SC1_3P3 (I/O), IO1_V_PD_ON_5P_SC1_3P3 (I/O), IO1_V_PU_ON_5P_!SC1_3P3 (I/O), IO1_V_PUPDOFF_5P_!SC1_3P3 (I/O), IO1_V_PU_ON_5P_SC1_3P3 (I/O), IO1_V_PUPDOFF_10P_SC1_1P8 (I/O), IO1_V_PD_ON_10P_!SC1_1P8 (I/O), IO1_V_PD_ON_10P_SC1_1P8 (I/O), IO1_V_PU_ON_10P_!SC1_1P8 (I/O), IO1_V_PUPDOFF_10P_!SC1_1P8 (I/O), IO1_V_PU_ON_10P_SC1_1P8 (I/O), IO1_V_PUPDOFF_10P_SC1_3P3 (I/O), IO1_V_PD_ON_10P_!SC1_3P3 (I/O), IO1_V_PD_ON_10P_SC1_3P3 (I/O), IO1_V_PU_ON_10P_!SC1_3P3 (I/O), IO1_V_PUPDOFF_10P_!SC1_3P3 (I/O), IO1_V_PU_ON_10P_SC1_3P3 (I/O), IO2_H_PUPDOFF_5P_SC1_1P8 (I/O), IO2_H_PD_ON_5P_!SC1_1P8 (I/O), IO2_H_PD_ON_5P_SC1_1P8 (I/O), IO2_H_PU_ON_5P_!SC1_1P8 (I/O), IO2_H_PUPDOFF_5P_!SC1_1P8 (I/O), IO2_H_PU_ON_5P_SC1_1P8 (I/O), IO2_H_PUPDOFF_5P_SC1_3P3 (I/O), IO2_H_PD_ON_5P_!SC1_3P3 (I/O), IO2_H_PD_ON_5P_SC1_3P3 (I/O), IO2_H_PU_ON_5P_!SC1_3P3 (I/O), IO2_H_PUPDOFF_5P_!SC1_3P3 (I/O), IO2_H_PU_ON_5P_SC1_3P3 (I/O), IO2_H_PUPDOFF_10P_SC1_1P8 (I/O), IO2_H_PD_ON_10P_!SC1_1P8 (I/O), IO2_H_PD_ON_10P_SC1_1P8 (I/O), IO2_H_PU_ON_10P_!SC1_1P8 (I/O), IO2_H_PUPDOFF_10P_!SC1_1P8 (I/O), IO2_H_PU_ON_10P_SC1_1P8 (I/O), IO2_H_PUPDOFF_10P_SC1_3P3 (I/O), IO2_H_PD_ON_10P_!SC1_3P3 (I/O), IO2_H_PD_ON_10P_SC1_3P3 (I/O), IO2_H_PU_ON_10P_!SC1_3P3 (I/O), IO2_H_PUPDOFF_10P_!SC1_3P3 (I/O), IO2_H_PU_ON_10P_SC1_3P3 (I/O), ODF_ADDON_HSTX (Output), ODF_ADDON_LPCD (Input), ODF_ADDON_LPRX (Input), ODF_ADDON_LPTX (Output), ODF_ADDON_ULPRX (Input), ODF_CORE_HSTX (Output), ODF_CORE_LPCD (Input), ODF_CORE_LPRX (Input)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
